(* Logix 5000 AddOnInstructionDefinition export Banner_CL50Pro_PD_v4; software revision 33.00 *)

TYPE Banner_CL50Pro_PDO_v4 :   // UDT that records the converted prcoess data.
STRUCT
   Color1 : SINT;   // 0 = Green, 1 = Red, 2 = Orange, 3 = Amber, 4 = Yellow, 5 = Lime Green, 6 = Spring Green, 7 = Cyan, 8 = SKy Blue, 9 = Blue, 10 = Violet, 11 = Magenta, 12 = Rose, 13 = White, 14 Custom 1, 15 = Custom 2.
   Color2 : SINT;   // 0 = Green, 1 = Red, 2 = Orange, 3 = Amber, 4 = Yellow, 5 = Lime Green, 6 = Spring Green, 7 = Cyan, 8 = SKy Blue, 9 = Blue, 10 = Violet, 11 = Magenta, 12 = Rose, 13 = White, 14 Custom 1, 15 = Custom 2.
   Animation : SINT;   // 0 = Off, 1 = Steady, 2 = Flash, 3 = Two Color Flash, 5 = Intensity Sweep
   Pulse_Pattern : SINT;   // 0 = Normal, 1 = Strobe, 2 = Three Pulse, 3 = SOS, 4 = Random
   Speed : SINT;   // 0 = Medium, 1 = Fast, 2 = Slow
   Color1_Intensity : SINT;   // 0 = High, 1 = Low, 2 = Medium, 3 = Off, 4 = Custom
   Color2_Intensity : SINT;   // 0 = High, 1 = Low, 2 = Medium, 3 = Off, 4 = Custom
   Audible_State : SINT;   // 0 = Off, 1 = On, 2 = Pulsed, 3 = SOS Pulse
   PDO_DT : SINT[4];
END_STRUCT
END_TYPE

ADD_ON_INSTRUCTION Banner_CL50Pro_PD_v4   (* revision 4.0, vendor Banner Engineering *)
// Takes the raw SINT information and converts that data into actual information.
VAR_IN_OUT
   Process_Data : Banner_CL50Pro_PDO_v4; {required}
END_VAR
VAR_INPUT
   Byte_Swap : BOOL; {required}
END_VAR
VAR
   PDO_Temp : SINT[10]; {access None}
   PDI_Temp : SINT[2]; {access None}
END_VAR

ROUTINE Logic   (* ladder *)
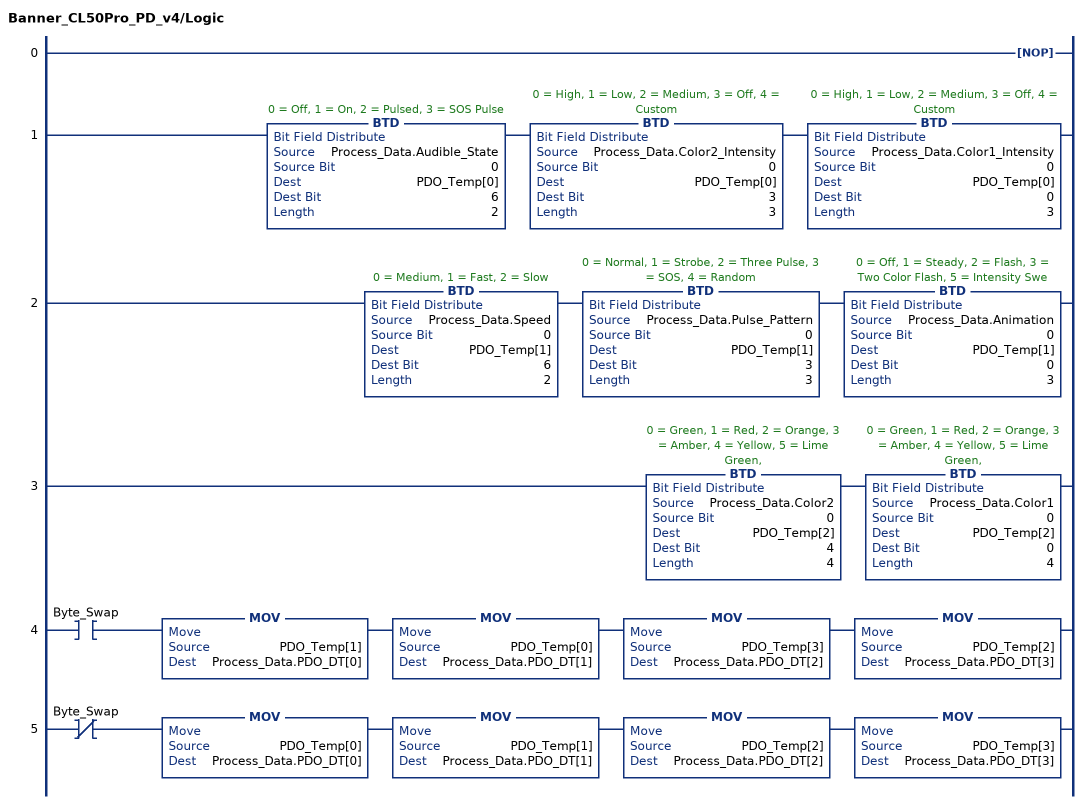
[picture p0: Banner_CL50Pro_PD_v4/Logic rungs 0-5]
   0: NOP();
   1: BTD(Process_Data.Audible_State,0,PDO_Temp[0],6,2)BTD(Process_Data.Color2_Intensity,0,PDO_Temp[0],3,3)BTD(Process_Data.Color1_Intensity,0,PDO_Temp[0],0,3);
   2: BTD(Process_Data.Speed,0,PDO_Temp[1],6,2)BTD(Process_Data.Pulse_Pattern,0,PDO_Temp[1],3,3)BTD(Process_Data.Animation,0,PDO_Temp[1],0,3);
   3: BTD(Process_Data.Color2,0,PDO_Temp[2],4,4)BTD(Process_Data.Color1,0,PDO_Temp[2],0,4);
   4: XIC(Byte_Swap)MOV(PDO_Temp[1],Process_Data.PDO_DT[0])MOV(PDO_Temp[0],Process_Data.PDO_DT[1])MOV(PDO_Temp[3],Process_Data.PDO_DT[2])MOV(PDO_Temp[2],Process_Data.PDO_DT[3]);
   5: XIO(Byte_Swap)MOV(PDO_Temp[0],Process_Data.PDO_DT[0])MOV(PDO_Temp[1],Process_Data.PDO_DT[1])MOV(PDO_Temp[2],Process_Data.PDO_DT[2])MOV(PDO_Temp[3],Process_Data.PDO_DT[3]);
END_ROUTINE
END_ADD_ON_INSTRUCTION
